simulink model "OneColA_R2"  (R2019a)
settings: Solver=ode15s  StartTime=0.0  StopTime=tend  RelTol=1e-3
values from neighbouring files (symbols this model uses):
  Extract_J = zeros(83,1)'    [Simulate1Col.m]    (also in Simulate1Col_OL.m; Simulate1Col_R1.m; Simulate1Col_R2.m)
  Extract_xB = zeros(82,1)'    [Simulate1Col.m]    (also in Simulate1Col_OL.m; Simulate1Col_R1.m; Simulate1Col_R2.m)
  Extract_xD = zeros(82,1)'    [Simulate1Col.m]    (also in Simulate1Col_OL.m; Simulate1Col_R1.m; Simulate1Col_R2.m)
  F0 = 1    [colamod.m]    (also in ColumnA_simulation.m; Simulate1Col.m = F; Simulate1Col_OL.m = F; Simulate1Col_R1.m = F)
  F0step = 0.05    [Simulate1Col.m]    (also in Simulate1Col_OL.m = 1*F0*.1; Simulate1Col_R1.m; Simulate1Col_R2.m = 0.15)
  F0step2 = 0*(0.15-F0step)    (= 0)    [Simulate1Col.m]    (also in Simulate1Col_R1.m; Simulate1Col_R2.m = 0.1)
  F0step2_t = 30    [Simulate1Col.m]    (also in Simulate1Col_R1.m; Simulate1Col_R2.m = 80)
  F0step_t = 10    [Simulate1Col.m]    (also in Simulate1Col_OL.m; Simulate1Col_R1.m; Simulate1Col_R2.m)
  Fbias = Fmax    (= 1.6825)    [Simulate1Col_R2.m]
  Kc_FxD = tau_FxD /(K_FxD *(tauc_FxD+theta_FxD))    (= -1.50442477876)    [TuningCol.m]
  Kc_LTxD = tau_LTxD /(K_LTxD *(tauc_LTxD+theta_LTxD))    (= 23.0752764867)    [TuningCol.m]
  Kc_VxB = tau_VxB /(K_VxB *(tauc_VxB+theta_VxB))    (= 83.8414634146)    [TuningCol.m]
  KI_FxD = Kc_FxD/tauI_FxD    [TuningCol.m]
  KI_LTxD = Kc_LTxD/tauI_LTxD    [TuningCol.m]
  KI_VxB = Kc_VxB/tauI_VxB    [TuningCol.m]
  LmaxPI = Lmax-LT0    [Simulate1Col.m]    (also in Simulate1Col_R1.m; Simulate1Col_R2.m)
  LT0 = u_opt(1)    [Simulate1Col.m]    (also in Simulate1Col_OL.m; Simulate1Col_R1.m; Simulate1Col_R2.m)
  pV0 = pV    [Simulate1Col.m]    (also in Simulate1Col_OL.m; Simulate1Col_R1.m; Simulate1Col_R2.m)
  pVstep = 0.02    [Simulate1Col.m]    (also in Simulate1Col_OL.m = 0*(0.13-pV0); Simulate1Col_R1.m; Simulate1Col_R2.m = 0.06)
  pVstept = 50    [Simulate1Col.m]    (also in Simulate1Col_OL.m; Simulate1Col_R1.m; Simulate1Col_R2.m)
  qF = U(7)    [colamod.m]    (also in ColumnA_simulation.m; Simulate1Col.m = 1; Simulate1Col_OL.m = 1; Simulate1Col_R1.m = 1)
  VB0 = u_opt(2)    [Simulate1Col.m]    (also in Simulate1Col_OL.m; Simulate1Col_R1.m; Simulate1Col_R2.m)
  VmaxPI = Vmax-VB0    [Simulate1Col.m]    (also in Simulate1Col_R1.m; Simulate1Col_R2.m)
  x0 = 0.5*ones(1,82)'    [col_obj.m]    (also in Simulate1Col.m = x; Simulate1Col_OL.m = x; Simulate1Col_R1.m = x; Simulate1Col_R2.m = x)
  xBsp = 0.95    [Simulate1Col.m]    (also in Simulate1Col_OL.m; Simulate1Col_R1.m; Simulate1Col_R2.m)
  xDmin = 0.95    [Simulate1Col.m]    (also in Simulate1Col_OL.m; Simulate1Col_R1.m; Simulate1Col_R2.m)
  zF = U(6)    [colamod.m]    (also in ColumnA_simulation.m; Simulate1Col.m = 0.5; Simulate1Col_OL.m = 0.5; Simulate1Col_R1.m = 0.5)
undefined symbols (not defined in the file or in its folder): Calc_xDsp, ColumnA_simulation, extract, LVMassBalance
libraries: simulink x3

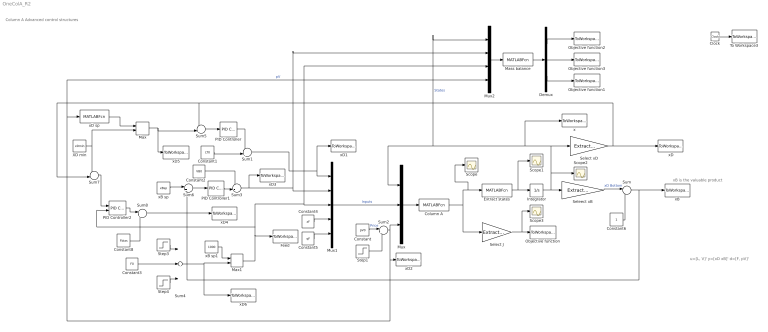
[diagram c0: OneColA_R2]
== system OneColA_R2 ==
  note: u=[L, V]' y=[xD xB]' d=[F, pV]'
  note: xB is the valuable product
  note: Column A Advanced control structures
  Clock : Clock
  Column A : MATLABFcn  MATLABFcn=ColumnA_simulation(u)  OutputDimensions=83
  Constant : Constant  Value=pV0
  Constant1 : Constant  Value=LT0
  Constant2 : Constant  Value=VB0
  Constant3 : Constant  Value=F0
  Constant4 : Constant  Value=zF
  Constant5 : Constant  Value=qF
  Constant6 : Constant
  Constant8 : Constant  Value=Fbias
  Demux : Demux  Outputs=3
  Extract states : MATLABFcn  MATLABFcn=extract(u)  OutputDimensions=82
  Feed : ToWorkspace  VariableName=Fin  SampleTime=-1
  Integrator : Integrator  InitialCondition=x0
  Mass balance : MATLABFcn  MATLABFcn=LVMassBalance(u)  OutputDimensions=3
  Max : MinMax  Function=max  Inputs=2
  Max1 : MinMax  Inputs=2
  Mux : Mux  Inputs=3
  Mux1 : Mux  Inputs=5
  Mux2 : Mux
  Objective function : ToWorkspace  VariableName=Jactual  SampleTime=-1
  Objective function1 : ToWorkspace  VariableName=Jreal  SampleTime=-1
  Objective function2 : ToWorkspace  VariableName=Dcurrent  SampleTime=-1
  Objective function3 : ToWorkspace  VariableName=Bcurrent  SampleTime=-1
  PID Controller : simulink/Continuous/PID Controller  Controller=PI  Form=Parallel  TimeDomain=Continuous-time  SampleTime=-1  IntegratorMethod=Forward Euler  FilterMethod=Forward Euler  ControllerParametersSource=internal  P=Kc_LTxD  I=KI_LTxD  D=0  UseFilter=on  N=100  TunerSelectOption=Transfer Function Based (PID Tuner App)  InitialConditionSource=internal  InitialConditionForIntegrator=0  InitialConditionForFilter=0  DifferentiatorICPrevScaledInput=0  ExternalReset=none  TrackingMode=off  Kt=1  LimitOutput=on  UpperSaturationLimit=LmaxPI  LowerSaturationLimit=-LT0  LinearizeAsGain=on  AntiWindupMode=none  Kb=1  POutMin=[]  POutMax=[]  IOutMin=[]  IOutMax=[]  DOutMin=[]  DOutMax=[]  NOutMin=[]  NOutMax=[]  SumOutMin=[]  SumOutMax=[]  SaturationOutMin=[]  SaturationOutMax=[]  PParamMin=[]  PParamMax=[]  IParamMin=[]  IParamMax=[]  DParamMin=[]  DParamMax=[]  NParamMin=[]  NParamMax=[]  KbParamMin=[]  KbParamMax=[]  KtParamMin=[]  KtParamMax=[]  KbOutMin=[]  KbOutMax=[]  KtOutMin=[]  KtOutMax=[]  IntegratorOutMin=[]  IntegratorOutMax=[]  FilterOutMin=[]  FilterOutMax=[]  SumI1OutMin=[]  SumI1OutMax=[]  SumI2OutMin=[]  SumI2OutMax=[]  SumI3OutMin=[]  SumI3OutMax=[]  SumI4OutMin=[]  SumI4OutMax=[]  SumDOutMin=[]  SumDOutMax=[]  DifferentiatorOutMin=[]  DifferentiatorOutMax=[]  FilterDiffOutCoefMin=[]  FilterDiffOutCoefMax=[]  ReciprocalOutMin=[]  ReciprocalOutMax=[]  SumDenOutMin=[]  SumDenOutMax=[]  SumNumOutMin=[]  SumNumOutMax=[]  DivideOutMin=[]  DivideOutMax=[]  IntegratorContinuousStateAttributes=''  IntegratorStateMustResolveToSignalObject=off  IntegratorRTWStateStorageClass=Auto  FilterContinuousStateAttributes=''  FilterStateMustResolveToSignalObject=off  FilterRTWStateStorageClass=Auto  ParallelPVariant=InternalParameters  IdealPVariant=Disabled  IVariant=InternalParameters  DVariant=Disabled  IntegratorVariant=Continuous  SatVariant=Enabled  AWVariant=Passthrough  PCopyVariant=Disabled  TRVariant=Disabled  FdbkBlocksVariant=Forward  IdealPFdbkVariant=Disabled  SatFdbkVariant=Disabled  DerivativeFilterVariant=Disabled  NVariant=Disabled  NCopyVariant=Disabled_SignalSpec  FilterICVariant=Disabled  IntegratorICVariant=InternalICs  ExternalResetVariant=Disabled  TRSumVariant=Passthrough  SumFdbkVariant=Disabled  SumVariant=Sum_PI
  PID Controller1 : simulink/Continuous/PID Controller  Controller=PI  Form=Parallel  TimeDomain=Continuous-time  SampleTime=-1  IntegratorMethod=Forward Euler  FilterMethod=Forward Euler  ControllerParametersSource=internal  P=Kc_VxB  I=KI_VxB  D=0  UseFilter=on  N=100  TunerSelectOption=Transfer Function Based (PID Tuner App)  InitialConditionSource=internal  InitialConditionForIntegrator=0  InitialConditionForFilter=0  DifferentiatorICPrevScaledInput=0  ExternalReset=none  TrackingMode=off  Kt=1  LimitOutput=on  UpperSaturationLimit=VmaxPI  LowerSaturationLimit=-VB0  LinearizeAsGain=on  AntiWindupMode=none  Kb=1  POutMin=[]  POutMax=[]  IOutMin=[]  IOutMax=[]  DOutMin=[]  DOutMax=[]  NOutMin=[]  NOutMax=[]  SumOutMin=[]  SumOutMax=[]  SaturationOutMin=[]  SaturationOutMax=[]  PParamMin=[]  PParamMax=[]  IParamMin=[]  IParamMax=[]  DParamMin=[]  DParamMax=[]  NParamMin=[]  NParamMax=[]  KbParamMin=[]  KbParamMax=[]  KtParamMin=[]  KtParamMax=[]  KbOutMin=[]  KbOutMax=[]  KtOutMin=[]  KtOutMax=[]  IntegratorOutMin=[]  IntegratorOutMax=[]  FilterOutMin=[]  FilterOutMax=[]  SumI1OutMin=[]  SumI1OutMax=[]  SumI2OutMin=[]  SumI2OutMax=[]  SumI3OutMin=[]  SumI3OutMax=[]  SumI4OutMin=[]  SumI4OutMax=[]  SumDOutMin=[]  SumDOutMax=[]  DifferentiatorOutMin=[]  DifferentiatorOutMax=[]  FilterDiffOutCoefMin=[]  FilterDiffOutCoefMax=[]  ReciprocalOutMin=[]  ReciprocalOutMax=[]  SumDenOutMin=[]  SumDenOutMax=[]  SumNumOutMin=[]  SumNumOutMax=[]  DivideOutMin=[]  DivideOutMax=[]  IntegratorContinuousStateAttributes=''  IntegratorStateMustResolveToSignalObject=off  IntegratorRTWStateStorageClass=Auto  FilterContinuousStateAttributes=''  FilterStateMustResolveToSignalObject=off  FilterRTWStateStorageClass=Auto  ParallelPVariant=InternalParameters  IdealPVariant=Disabled  IVariant=InternalParameters  DVariant=Disabled  IntegratorVariant=Continuous  SatVariant=Enabled  AWVariant=Passthrough  PCopyVariant=Disabled  TRVariant=Disabled  FdbkBlocksVariant=Forward  IdealPFdbkVariant=Disabled  SatFdbkVariant=Disabled  DerivativeFilterVariant=Disabled  NVariant=Disabled  NCopyVariant=Disabled_SignalSpec  FilterICVariant=Disabled  IntegratorICVariant=InternalICs  ExternalResetVariant=Disabled  TRSumVariant=Passthrough  SumFdbkVariant=Disabled  SumVariant=Sum_PI
  PID Controller2 : simulink/Continuous/PID Controller  Controller=PI  Form=Parallel  TimeDomain=Continuous-time  SampleTime=-1  IntegratorMethod=Forward Euler  FilterMethod=Forward Euler  ControllerParametersSource=internal  P=Kc_FxD  I=KI_FxD  D=0  UseFilter=on  N=100  TunerSelectOption=Transfer Function Based (PID Tuner App)  InitialConditionSource=internal  InitialConditionForIntegrator=0  InitialConditionForFilter=0  DifferentiatorICPrevScaledInput=0  ExternalReset=none  TrackingMode=on  Kt=1  LimitOutput=off  UpperSaturationLimit=VmaxPI  LowerSaturationLimit=-VB0  LinearizeAsGain=on  AntiWindupMode=none  Kb=1  POutMin=[]  POutMax=[]  IOutMin=[]  IOutMax=[]  DOutMin=[]  DOutMax=[]  NOutMin=[]  NOutMax=[]  SumOutMin=[]  SumOutMax=[]  SaturationOutMin=[]  SaturationOutMax=[]  PParamMin=[]  PParamMax=[]  IParamMin=[]  IParamMax=[]  DParamMin=[]  DParamMax=[]  NParamMin=[]  NParamMax=[]  KbParamMin=[]  KbParamMax=[]  KtParamMin=[]  KtParamMax=[]  KbOutMin=[]  KbOutMax=[]  KtOutMin=[]  KtOutMax=[]  IntegratorOutMin=[]  IntegratorOutMax=[]  FilterOutMin=[]  FilterOutMax=[]  SumI1OutMin=[]  SumI1OutMax=[]  SumI2OutMin=[]  SumI2OutMax=[]  SumI3OutMin=[]  SumI3OutMax=[]  SumI4OutMin=[]  SumI4OutMax=[]  SumDOutMin=[]  SumDOutMax=[]  DifferentiatorOutMin=[]  DifferentiatorOutMax=[]  FilterDiffOutCoefMin=[]  FilterDiffOutCoefMax=[]  ReciprocalOutMin=[]  ReciprocalOutMax=[]  SumDenOutMin=[]  SumDenOutMax=[]  SumNumOutMin=[]  SumNumOutMax=[]  DivideOutMin=[]  DivideOutMax=[]  IntegratorContinuousStateAttributes=''  IntegratorStateMustResolveToSignalObject=off  IntegratorRTWStateStorageClass=Auto  FilterContinuousStateAttributes=''  FilterStateMustResolveToSignalObject=off  FilterRTWStateStorageClass=Auto  ParallelPVariant=InternalParameters  IdealPVariant=Disabled  IVariant=InternalParameters  DVariant=Disabled  IntegratorVariant=Continuous  SatVariant=Disabled  AWVariant=Passthrough  PCopyVariant=Disabled  TRVariant=Enabled  FdbkBlocksVariant=Forward  IdealPFdbkVariant=Disabled  SatFdbkVariant=Disabled  DerivativeFilterVariant=Disabled  NVariant=Disabled  NCopyVariant=Disabled_SignalSpec  FilterICVariant=Disabled  IntegratorICVariant=InternalICs  ExternalResetVariant=Disabled  TRSumVariant=TrackingMode  SumFdbkVariant=Disabled  SumVariant=Sum_PI
  Scope{,1..3} (4 alike) : Scope
  Select J : Gain  Gain=Extract_J  Multiplication=Matrix(K*u)
  Select xD : Gain  Gain=Extract_xD  Multiplication=Matrix(K*u)
  Seleect xB : Gain  Gain=Extract_xB  Multiplication=Matrix(K*u)
  Step1 : Step  Time=pVstept  After=pVstep  SampleTime=0
  Step3 : Step  Time=F0step_t  After=F0step  SampleTime=0
  Step4 : Step  Time=F0step2_t  After=F0step2  SampleTime=0
  Sum : Sum  Inputs=|-+
  Sum1 : Sum  Inputs=++|
  Sum2 : Sum  Inputs=|++
  Sum3 : Sum  Inputs=++|
  Sum4 : Sum  Inputs=+++
  Sum5 : Sum  Inputs=-+|
  Sum6 : Sum  Inputs=|+-
  Sum7 : Sum  Inputs=+-|
  Sum8 : Sum  Inputs=|++
  To Workspace3 : ToWorkspace  VariableName=time  SampleTime=-1
  XD min : Constant  Value=xDmin
  x : ToWorkspace  VariableName=States  SampleTime=-1
  xB : ToWorkspace  VariableName=xB  SampleTime=-1
  xB sp : Constant  Value=xBsp
  xB sp1 : Constant  Value=1000
  xD : ToWorkspace  VariableName=xD  SampleTime=-1
  xD sp : MATLABFcn  MATLABFcn=Calc_xDsp(u)  OutputDimensions=1
  xD1 : ToWorkspace  VariableName=LT  SampleTime=-1
  xD2 : ToWorkspace  VariableName=pV  SampleTime=-1
  xD3 : ToWorkspace  VariableName=VB  SampleTime=-1
  xD4 : ToWorkspace  VariableName=Fin_xD  SampleTime=-1
  xD5 : ToWorkspace  VariableName=xDsp  SampleTime=-1
  xD6 : ToWorkspace  VariableName=Fin_sp  SampleTime=-1
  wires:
  Mux/1 -> Column A/1
  Mux1/1 -> Mux/2  "Inputs"
  Constant4/1 -> Mux1/4
  Constant5/1 -> Mux1/5
  Column A/1 -> Select J/1, Extract states/1, Scope/1
  Extract states/1 -> Scope1/1, Integrator/1
  Integrator/1 -> Seleect xB/1, Select xD/1, x/1, Mux2/1, Mux/1, Scope2/1  "States"
  Select xD/1 -> Sum7/2, Sum5/1, xD/1
  Select J/1 -> Scope3/1, Objective function/1
  Clock/1 -> To Workspace3/1
  Seleect xB/1 -> Sum/1  "xD Bottom"
  Sum/1 -> xB/1, Sum6/2
  Constant6/1 -> Sum/2
  Sum1/1 -> xD1/1, Mux1/1
  Sum2/1 -> xD2/1, Mux2/4, xD sp/1, Mux/3  "pV"
  Constant/1 -> Sum2/1  "Price"
  Sum3/1 -> Mux2/2, Mux1/2, xD3/1
  Step1/1 -> Sum2/2
  Sum5/1 -> PID Controller/1
  Constant2/1 -> Sum3/1
  Constant1/1 -> Sum1/2
  PID Controller1/1 -> Sum3/2
  Sum6/1 -> PID Controller1/1
  xB sp/1 -> Sum6/1
  Max/1 -> xD5/1, Sum5/2
  xD sp/1 -> Max/1
  XD min/1 -> Max/2, Sum7/1
  Constant3/1 -> Sum4/2
  Step4/1 -> Sum4/3
  Step3/1 -> Sum4/1
  Max1/1 -> Mux2/3, Mux1/3, PID Controller2/2, Feed/1
  Sum7/1 -> PID Controller2/1
  Sum4/1 -> xD6/1, Max1/2
  Sum8/1 -> xD4/1
  PID Controller2/1 -> Sum8/1
  Constant8/1 -> Sum8/2
  xB sp1/1 -> Max1/1
  PID Controller/1 -> Sum1/1
  Mass balance/1 -> Demux/1
  Demux/3 -> Objective function1/1
  Mux2/1 -> Mass balance/1
  Demux/1 -> Objective function2/1
  Demux/2 -> Objective function3/1
